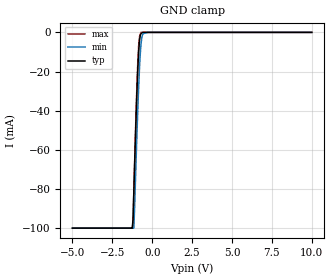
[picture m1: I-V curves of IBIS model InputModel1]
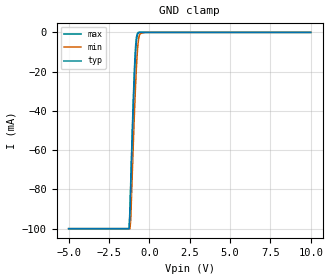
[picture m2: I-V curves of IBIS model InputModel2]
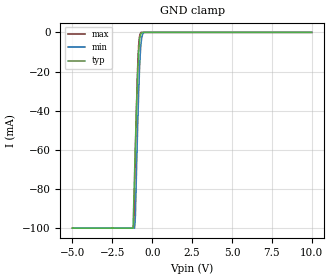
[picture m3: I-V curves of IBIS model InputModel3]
[IBIS Ver]   2.1
[File name]   pa002bc5.ibs   | e_= PSOP, f002bc= abbr chip name, 5 = 5V Vcc
[File Rev]   2.00
[Date]   3-April-96
[Source]   File generated from lab measurements at Intel Corporation
[Notes]   This model is for both the 28F002BC-T & 28F002BC-B.
   Rev 2.00 All data was replaced by actual measurements
   performed in a lab.
[Disclaimer] INTEL DEVELOPER'S SOFTWARE LICENSE AGREEMENT
| BY USING THIS SOFTWARE, YOU ARE AGREEING TO BE BOUND
| BY THE TERMS OFTHIS AGREEMENT.  DO NOT USE THE SOFTWARE
| UNTIL YOU HAVE CAREFULLY READAND AGREED TO THE FOLLOWING
| TERMS AND CONDITIONS.  IF YOU DO NOT AGREETO THE TERMS
| OF THIS AGREEMENT, PROMPTLY RETURN THE SOFTWARE PACKAGE
| ANDANY ACCOMPANYING ITEMS.
| IF YOU USE THIS SOFTWARE, YOU WILL BE BOUND BY THE TERMS
| OF THIS AGREEMENT
| LICENSE: Intel Corporation ("Intel") grants you the non-exclusive right
| to use the enclosed software program ("Software").  You will not use,
| copy, modify, rent, sell or transfer the Software or any portion
| thereof, except as provided in this Agreement.
| System OEM Developers may:
| 1.   Copy the Software for support, backup or archival purposes;
| 2.   Install, use, or distribute Intel owned Software in object code
|   only;
| 3.   Modify and/or use Software source code that Intel directly makes
|   available to you as an OEM Developer;
| 4.   Install, use, modify, distribute, and/or make or have made
|   derivatives ("Derivatives") of Intel owned Software under the
|   terms and conditions in this Agreement, ONLY if you are a System
|   OEM Developer and NOT an end-user.
| RESTRICTIONS:
| YOU WILL NOT:
| 1.   Copy the Software, in whole or in part, except as provided for
|   in this Agreement;
| 2.   Decompile or reverse engineer any Software provided in object
|   code format;
| 3.   Distribute any Software or Derivative code to any end-users,
|   unless approved by Intel in a prior writing.
| TRANSFER: You may transfer the Software to another OEM
| Developer if thereceiving party agrees to the terms of this
| Agreement at the sole risk of any receiving party.
| OWNERSHIP AND COPYRIGHT OF SOFTWARE:
| Title to the Software and all copies thereof remain with Intel
| or its vendors.  The Software iscopyrighted and is protected by
| United States and international copyright laws.  You will not
| remove the copyright notice from the Software.  You agree to
| prevent any unauthorized copying of the Software.
| DERIVATIVE WORK: OEM Developers that make or have made
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[Copyright]   Copyright 1996, Intel Corporation, All Rights Reserved
[Component]   PA28F002BC   | 44-lead PSOP package, 28F002BC
[Manufacturer]  Intel   | Boot Block (tm)
|   | operating in 5V Vcc range
[Package]
R_pkg   145.5m   144.0m   147.0m
L_pkg   5.25nH   2.00nH   8.50nH
C_pkg   1.09pF   0.68pF   1.50pF
|*****************************Pin Definitions*****************************
[Pin]   signal_name   model_name   R_pin   L_pin   C_pin
 1   VPP   POWER
 2   DU   InputModel4
 3   NC   InputModel1
 4   A07   InputModel1
 5   A06   InputModel1
 6   A05   InputModel1
 7   A04   InputModel1
 8   A03   InputModel1
 9   A02   InputModel1
10   A01   InputModel1
11   A00   InputModel2
12   CE#   InputModel3
13   GND   GND
14   OE#   InputModel3
15   DQ0   InputOutput
16   NC   InputModel4
17   DQ1   InputOutput
18   NC   InputModel4
19   DQ2   InputOutput
20   NC   InputModel4
21   DQ3   InputOutput
22   NC   InputModel4
23   VCC   POWER
24   DQ4   InputOutput
25   NC   InputModel4
26   DQ5   InputOutput
27   NC   InputModel4
28   DQ6   InputOutput
29   NC   InputModel4
30   DQ7   InputOutput
31   A-1   InputModel2
32   GND   GND
33   NC   InputModel4
34   A16   InputModel2
35   A15   InputModel1
36   A14   InputModel1
37   A13   InputModel1
38   A12   InputModel1
39   A11   InputModel1
40   A10   InputModel1
41   A09   InputModel1
42   A08   InputModel1
43   WE#   InputModel3
44   RP#   InputModel3
|***********************Input Model 4******************************
[Model]   InputModel4
Model_type   Input
|   Model for  DU & NC pins, excluding Pin #3.
Vinl = 0.8V
Vinh = 2.0V
|Variable   Typ   Min   Max
C_comp   5.61p   NA   7.6p
[Voltage Range]   5.0V   4.5V   5.5V
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| Models and submodels in the file (5): InputModel1 (Input), InputModel2 (Input), InputModel3 (Input), InputModel4 (Input), InputOutput (I/O)
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|*********************Input Model 1************************************
[Model]   InputModel1
Model_type   Input
|   Model for A[8:15] A[1:7] & NC (pin 3).
Vinl = 0.8V
Vinh = 2.0V
|Variable   Typ   Min   Max
C_comp   5.61p   NA   7.6p
[Voltage Range]   5.0V   4.5V   5.5V
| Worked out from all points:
|   GND clamp passes 1 mA (typ) near -0.72 V on its own axis
[GND_clamp]
|Voltage  I(typ)   I(min)   I(max)
-5V       -100mA     -100mA     -100mA
-1.25V    -100mA     -100mA     -100mA
-1.2V     -95.3mA    -100mA     -96.97mA
-1.15V    -80.92mA   -100mA     -81.41mA
-1V       -40.48mA   -62.87mA   -37.82mA
-900mV    -18.21mA   -38.72mA   -14.64mA
-850mV    -10.1mA    -28.28mA   -6.908mA
-800mV    -4.427mA   -18.77mA   -2.472mA
-700mV    -589.5uA   -5.79mA    0A
-600mV    0A         -1.063mA   0A
-250mV    0A         0A         0A
10V       0A         0A         0A
[Power_clamp]
| Input buffer circuits of this product do not intrinsically
| require a [Power_clamp] definition.  This zero current
| [Power_clamp] table is provided for the compatibility with
| some IBIS parsers.
|Voltage  I(typ)   I(min)   I(max)
-5V       0A         0A         0A
0V        0A         0A         0A
5V        0A         0A         0A
10V       0A         0A         0A
|*********************Input Model 2******************************
[Model]   InputModel2
Model_type   Input
|   Model for A[0], A[16] & A[-1] pins.
Vinl = 0.8V
Vinh = 2.0V
|Variable   Typ   Min   Max
C_comp   5.61p   NA   7.6p
[Voltage Range]   5.0V   4.5V   5.5V
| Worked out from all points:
|   GND clamp passes 1 mA (typ) near -0.72 V on its own axis
[GND_clamp]
|Voltage  I(typ)   I(min)   I(max)
-5V       -100mA     -100mA     -100mA
-1.25V    -100mA     -100mA     -100mA
-1.2V     -92.25mA   -100mA     -89.48mA
-1.15V    -78.35mA   -95.31mA   -75.23mA
-1V       -39.26mA   -58.42mA   -35.27mA
-900mV    -17.72mA   -36.17mA   -13.9mA
-850mV    -9.851mA   -26.51mA   -6.694mA
-800mV    -4.349mA   -17.72mA   -2.426mA
-700mV    -587.2uA   -5.568mA   0A
-600mV    0A         -1.028mA   0A
-250mV    0A         0A         0A
10V       0A         0A         0A
[Power_clamp]
| Input buffer circuits of this product do not intrinsically
| require a [Power_clamp] definition.  This zero current
| [Power_clamp] table is provided for the compatibility with
| some IBIS parsers.
|Voltage  I(typ)   I(min)   I(max)
-5V       0A         0A         0A
0V        0A         0A         0A
5V        0A         0A         0A
10V       0A         0A         0A
|***********************Input Model 3******************************
[Model]   InputModel3
Model_type   Input
|   Model for WE#, WP#, RP#, OE# & CE# pin.
Vinl = 0.8V
Vinh = 2.0V
|Variable   Typ   Min   Max
C_comp   5.61p   NA   7.6p
[Voltage Range]   5.0V   4.5V   5.5V
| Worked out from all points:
|   GND clamp passes 1 mA (typ) near -0.72 V on its own axis
[GND_clamp]
|Voltage  I(typ)   I(min)   I(max)
-5V       -100mA     -100mA     -100mA
-1.2V     -100mA     -100mA     -100mA
-1.15V    -85.5mA    -100mA     -98.31mA
-1.1V     -70.41mA   -100mA     -78.56mA
-1.05V    -56.02mA   -93.54mA   -59.94mA
-950mV    -29.73mA   -60.51mA   -27.3mA
-900mV    -18.71mA   -45.27mA   -14.84mA
-850mV    -10.25mA   -31.97mA   -6.48mA
-800mV    -4.452mA   -20.32mA   -2.166mA
-700mV    -580.8uA   -5.673mA   0A
-500mV    0A         0A         0A
10V       0A         0A         0A
[Power_clamp]
| Input buffer circuits of this product do not intrinsically
| require a [Power_clamp] definition.  This zero current
| [Power_clamp] table is provided for the compatibility with
| some IBIS parsers.
|Voltage  I(typ)   I(min)   I(max)
-5V       0A         0A         0A
0V        0A         0A         0A
5V        0A         0A         0A
10V       0A         0A         0A
